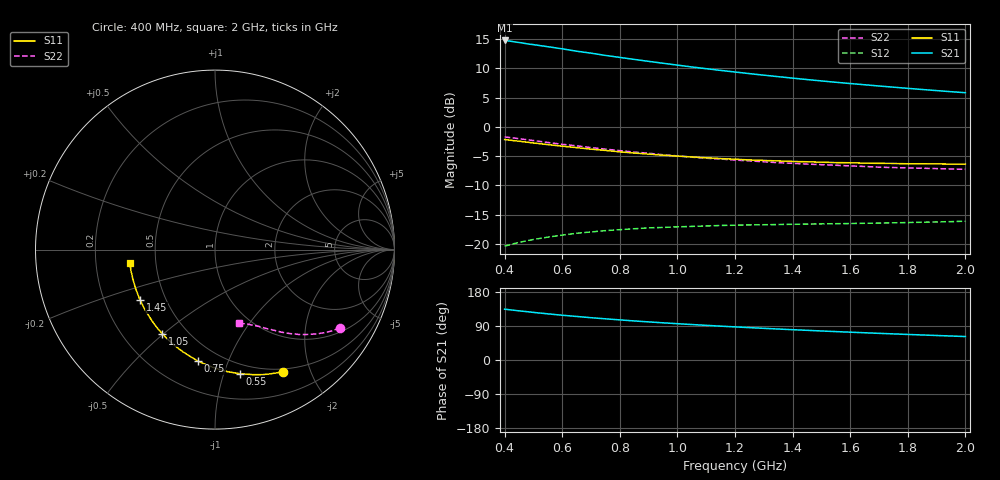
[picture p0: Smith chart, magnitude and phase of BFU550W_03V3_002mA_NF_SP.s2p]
! Filename:  P:\Prog\Test\Noise\ATS_data\Testdata_Net\06 Compressed Noise after Statistics\BFU550W_APM2013_11_D05_03p3V_002mA_NF_CM01_D.sf
! Date/Time: Tue 26/Mar/2013 16:25:28
! BFU550W_APM2013_11_D05_03p3V_1to35mA_NF_CM01_Bias2_R.sf
! Noise Parameter Data File
! BFU550W_APM2013_11_D05_03p3V_1to35mA_NF_CM01
! Date/time: Mon Mar 25 12:16:07 2013
! VAR V_out= 3.300000
! VAR I_out= 1.995000
! VAR V_in= 0.793300
! VAR I_in= 0.020600
! Device data file deembeded for feedlines and parallel
! Original file: \06 Compressed Noise after Statistics\BFU550W_APM2013_11_D05_03p3V_002mA_NF_CM01_R.sf
! Feed-files: PR019V01_070313_Feed1.s2p, PR019V01_070313_Feed2.s2p
! Parallel-file: PR019V01_070313_Par.s2p
# MHz S MA R 50
!  Freq-MHz  S11-mag  S11-arg  S21-mag  S21-arg  S12-mag  S12-arg  S22-mag  S22-arg
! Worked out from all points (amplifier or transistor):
!   37 points, 400 MHz to 2 GHz, reference 50 ohm
!   highest |S21| = 14.8 dB at 400 MHz (marker M1)
!   |S21| within 3 dB of that: start of sweep to 814.8 MHz
!   unconditionally stable (mu >= 1): nowhere
!   at 500 MHz: K = 0.29, MSG = 16.7 dB, |S12| = -19.3 dB
!   at 1.1 GHz: K = 0.60, MSG = 13.5 dB, |S12| = -17.0 dB
!   at 2 GHz: K = 0.97, MSG = 11.0 dB, |S12| = -16.1 dB
!   lowest NFmin = 0.48 dB at 420 MHz
!   S11 on the Smith chart (normalised r, x): 400 MHz: 0.46, -1.61; 550 MHz: 0.41, -1.13; 750 MHz: 0.38, -0.79; 1.05 GHz: 0.37, -0.49; 1.45 GHz: 0.36, -0.27; 2 GHz: 0.35, -0.07
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400  0.7793 -60.7  5.485 134.1  0.09539 56.6  0.8205 -32.1
420  0.7685 -63.4  5.407 132.3  0.09841 55.4  0.8093 -33.2
460  0.7488 -68.3  5.225 128.9  0.1039 53.2  0.7866 -35.4
480  0.7389 -70.6  5.125 127.3  0.1064 52.2  0.7752 -36.4
500  0.7283 -73.1  5.051 125.6  0.1088 51.2  0.7637 -37.3
550  0.705 -78.7  4.85 121.8  0.114 49.0  0.7355 -39.7
600  0.6836 -84.2  4.652 118.2  0.1187 47.0  0.7098 -41.7
650  0.6641 -89.0  4.439 114.9  0.123 45.2  0.6883 -43.4
700  0.6447 -94.1  4.271 111.6  0.1262 43.6  0.6649 -45.3
750  0.6287 -98.5  4.086 108.7  0.1295 42.2  0.6452 -46.7
800  0.6112 -103.0  3.929 105.8  0.1321 41.0  0.6263 -48.4
850  0.5972 -107.3  3.777 103.1  0.1344 39.9  0.6086 -49.6
950  0.5725 -115.1  3.502 98.1  0.1379 38.1  0.5773 -52.2
1050  0.5527 -122.2  3.255 93.6  0.1407 36.9  0.5508 -54.4
1150  0.5356 -129.1  3.041 89.3  0.1434 35.9  0.5312 -56.3
1200  0.5286 -132.0  2.946 87.3  0.144 35.7  0.52 -57.4
1300  0.5163 -138.1  2.769 83.6  0.1455 35.3  0.5026 -59.3
1450  0.503 -146.2  2.539 78.3  0.1473 35.4  0.4805 -61.9
1500  0.4987 -148.8  2.472 76.6  0.148 35.5  0.475 -62.8
1650  0.4895 -156.2  2.292 71.9  0.1497 36.3  0.4586 -65.4
1750  0.4864 -160.6  2.186 68.9  0.1511 37.2  0.4487 -67.1
2000  0.4808 -171.0  1.961 61.9  0.1559 39.9  0.4332 -71.7
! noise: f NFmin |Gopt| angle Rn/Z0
400  0.4922  0.4759  34.44  0.164
460  0.5055  0.4704  39.42  0.1689
600  0.5449  0.4912  45.2  0.1797
800  0.6104  0.4677  65.29  0.1459
1000  0.6598  0.4912  77.52  0.1474
1200  0.711  0.4819  92.41  0.1318
1400  0.7524  0.4726  108  0.1105
1600  0.7299  0.5014  123.4  0.0798
1800  0.8872  0.4812  135.7  0.0751
2000  0.9581  0.4885  147.8  0.0649
